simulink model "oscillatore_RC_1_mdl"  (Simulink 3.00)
settings: Solver=ode23s  StartTime=0.0  StopTime=10.0  RelTol=1e-6  AbsTol=1e-6
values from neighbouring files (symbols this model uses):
  C = 0.001    [oscillatore.m]    (also in oscillatore_RC.m; oscillatore_RC_1.m; oscillatore_wien.m)
  K = R1/(R1+R2)    (= 0.333333333333)    [oscillatore_RC.m]    (also in oscillatore_RC_1.m)
  Q30 = C*V30    (= 0.0001)    [oscillatore.m]    (also in oscillatore_RC.m; oscillatore_RC_1.m)
  R = 1    [oscillatore.m]    (also in oscillatore_RC.m; oscillatore_RC_1.m; oscillatore_wien.m)
  VM = 12    [oscillatore.m]    (also in oscillatore_RC.m; oscillatore_RC_1.m; oscillatore_wien.m)

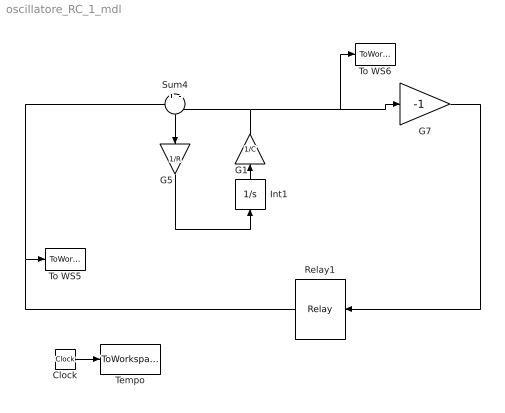
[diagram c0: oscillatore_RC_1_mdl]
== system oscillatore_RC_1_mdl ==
  Clock : Clock
  G1 : Gain  Orientation=up  Gain=1/C  SaturateOnIntegerOverflow=on
  G5 : Gain  Orientation=down  Gain=1/R  SaturateOnIntegerOverflow=on
  G7 : Gain  Gain=-1  SaturateOnIntegerOverflow=on
  Int1 : Integrator  Orientation=up  ExternalReset=none  InitialConditionSource=internal  InitialCondition=Q30  LimitOutput=off  UpperSaturationLimit=inf  LowerSaturationLimit=-inf  ShowSaturationPort=off  ShowStatePort=off  AbsoluteTolerance=auto
  Relay1 : Relay  Orientation=left  OnSwitchValue=VM*K  OffSwitchValue=-VM*K  OnOutputValue=VM  OffOutputValue=-VM
  Sum4 : Sum  Orientation=down  Inputs=+|-  SaturateOnIntegerOverflow=on
  Tempo : ToWorkspace  VariableName=t  SampleTime=-1  SaveFormat=Matrix
  To WS5 : ToWorkspace  VariableName=V0  SampleTime=-1  SaveFormat=Matrix
  To WS6 : ToWorkspace  VariableName=VP  SampleTime=-1  SaveFormat=Matrix
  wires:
  Clock/1 -> Tempo/1
  Relay1/1 -> To WS5/1, Sum4/1
  Int1/1 -> G1/1
  Sum4/1 -> G5/1
  G5/1 -> Int1/1
  G1/1 -> Sum4/2, G7/1, To WS6/1
  G7/1 -> Relay1/1
